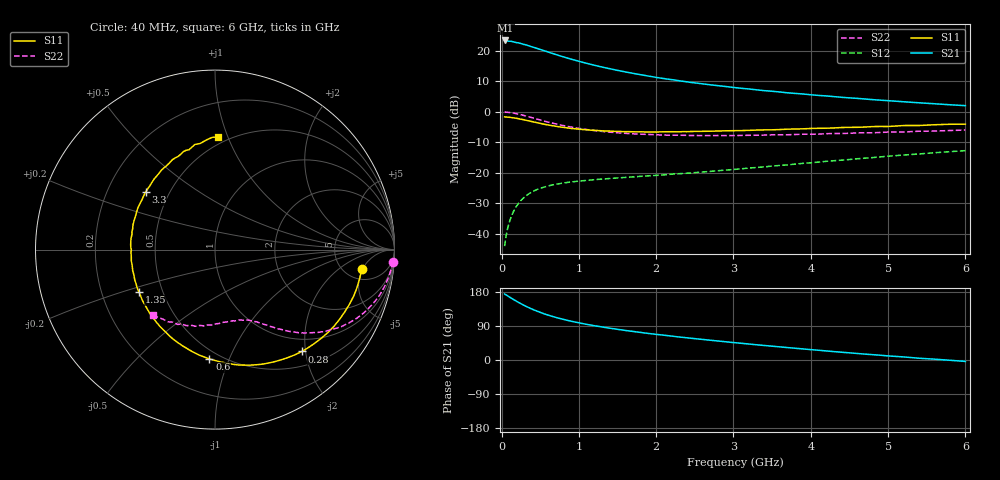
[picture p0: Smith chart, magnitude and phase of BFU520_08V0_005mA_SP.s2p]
! Filename:  P:\Prog\Test\Noise\ATS_data\Testdata_Net\03 Spar\BFU520_APG2013_37_A05_08p0V_005mA_SP_CM01_D.s2p
! Date/Time: Fri 26/Apr/2013 13:00:09
! BFU520_APG2013_37_A05_08p0V_1to20mA_SP_CM01_Bias4_R.s2p
! MDIF S-parameter v. bias file
! BFU520_APG2013_37_A05_08p0V_1to20mA_SP_CM01
! Date/time Tue Apr 23 17:06:44 2013
! VAR V_out= 8.0000
! VAR I_out= 5.0000
! VAR V_in= 0.8207
! VAR I_in= 0.0546
! Device data file deembeded for feedlines and parallel
! Original file: \03 Spar\BFU520_APG2013_37_A05_08p0V_005mA_SP_CM01_R.s2p
! Feed-files: PR047V01_250413_Feed1.s2p, PR047V01_250413_Feed2.s2p
! Parallel-file: PR047V01_250413_Par.s2p
# MHz S MA R 50
!  Freq-MHz  S11-mag  S11-arg  S21-mag  S21-arg  S12-mag  S12-arg  S22-mag  S22-arg
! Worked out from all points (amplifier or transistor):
!   98 points, 40 MHz to 6 GHz, reference 50 ohm
!   highest |S21| = 23.4 dB at 50 MHz (marker M1)
!   |S21| within 3 dB of that: start of sweep to 506.6 MHz
!   unconditionally stable (mu >= 1): 2.341 GHz to 4.349 GHz
!   at 300 MHz: K = 0.19, MSG = 25.0 dB, |S12| = -27.9 dB
!   at 1.6 GHz: K = 0.81, MSG = 17.3 dB, |S12| = -21.5 dB
!   at 6 GHz: K = 0.85, MSG = 7.4 dB, |S12| = -12.7 dB
!   S11 on the Smith chart (normalised r, x): 40 MHz: 7.18, -4.85; 280 MHz: 0.75, -1.93; 600 MHz: 0.44, -0.85; 1.35 GHz: 0.37, -0.23; 3.3 GHz: 0.37, +0.32; 6 GHz: 0.45, +0.93
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40  0.826 -7.5  14.79 174.3  0.006269 85.2  0.9915 -3.9
50  0.8239 -9.3  14.81 172.4  0.007829 84.7  0.99 -4.9
70  0.8202 -12.9  14.6 170.6  0.01088 82.8  0.9853 -7.0
120  0.8085 -22.2  14.37 163.9  0.01832 78.0  0.968 -11.9
160  0.7952 -29.3  13.99 159.1  0.02394 74.1  0.9507 -15.6
220  0.7711 -39.8  13.52 152.0  0.03156 69.1  0.9157 -20.9
280  0.7458 -49.5  12.82 145.5  0.03828 64.3  0.8781 -25.8
340  0.7165 -59.0  12.26 139.4  0.04402 60.4  0.8376 -29.9
420  0.6809 -70.5  11.38 132.2  0.05046 55.7  0.7849 -34.7
600  0.6097 -93.0  9.613 118.6  0.06076 48.1  0.6814 -43.0
700  0.5801 -103.4  8.731 112.5  0.06472 45.2  0.6348 -46.3
800  0.5561 -112.8  7.974 107.2  0.06807 43.1  0.5954 -49.1
1050  0.5122 -132.6  6.494 96.0  0.07413 39.8  0.5235 -54.6
1350  0.4853 -150.9  5.257 85.6  0.07976 38.4  0.4706 -59.4
1600  0.4729 -163.8  4.518 78.0  0.08402 38.3  0.4441 -63.2
2050  0.4695 178.3  3.588 66.6  0.09154 39.5  0.4183 -69.7
2450  0.4759 164.1  3.037 57.4  0.09942 41.0  0.4086 -75.9
3100  0.4929 145.4  2.436 44.1  0.1163 43.4  0.4106 -85.6
3300  0.5025 140.3  2.296 40.2  0.1223 43.7  0.413 -88.8
4100  0.5373 121.8  1.858 25.7  0.1498 43.7  0.4318 -101.8
5200  0.5962 100.8  1.463 8.2  0.1955 40.0  0.4677 -120.1
6000  0.6279 88.3  1.264 -3.7  0.2314 34.9  0.5026 -133.6
